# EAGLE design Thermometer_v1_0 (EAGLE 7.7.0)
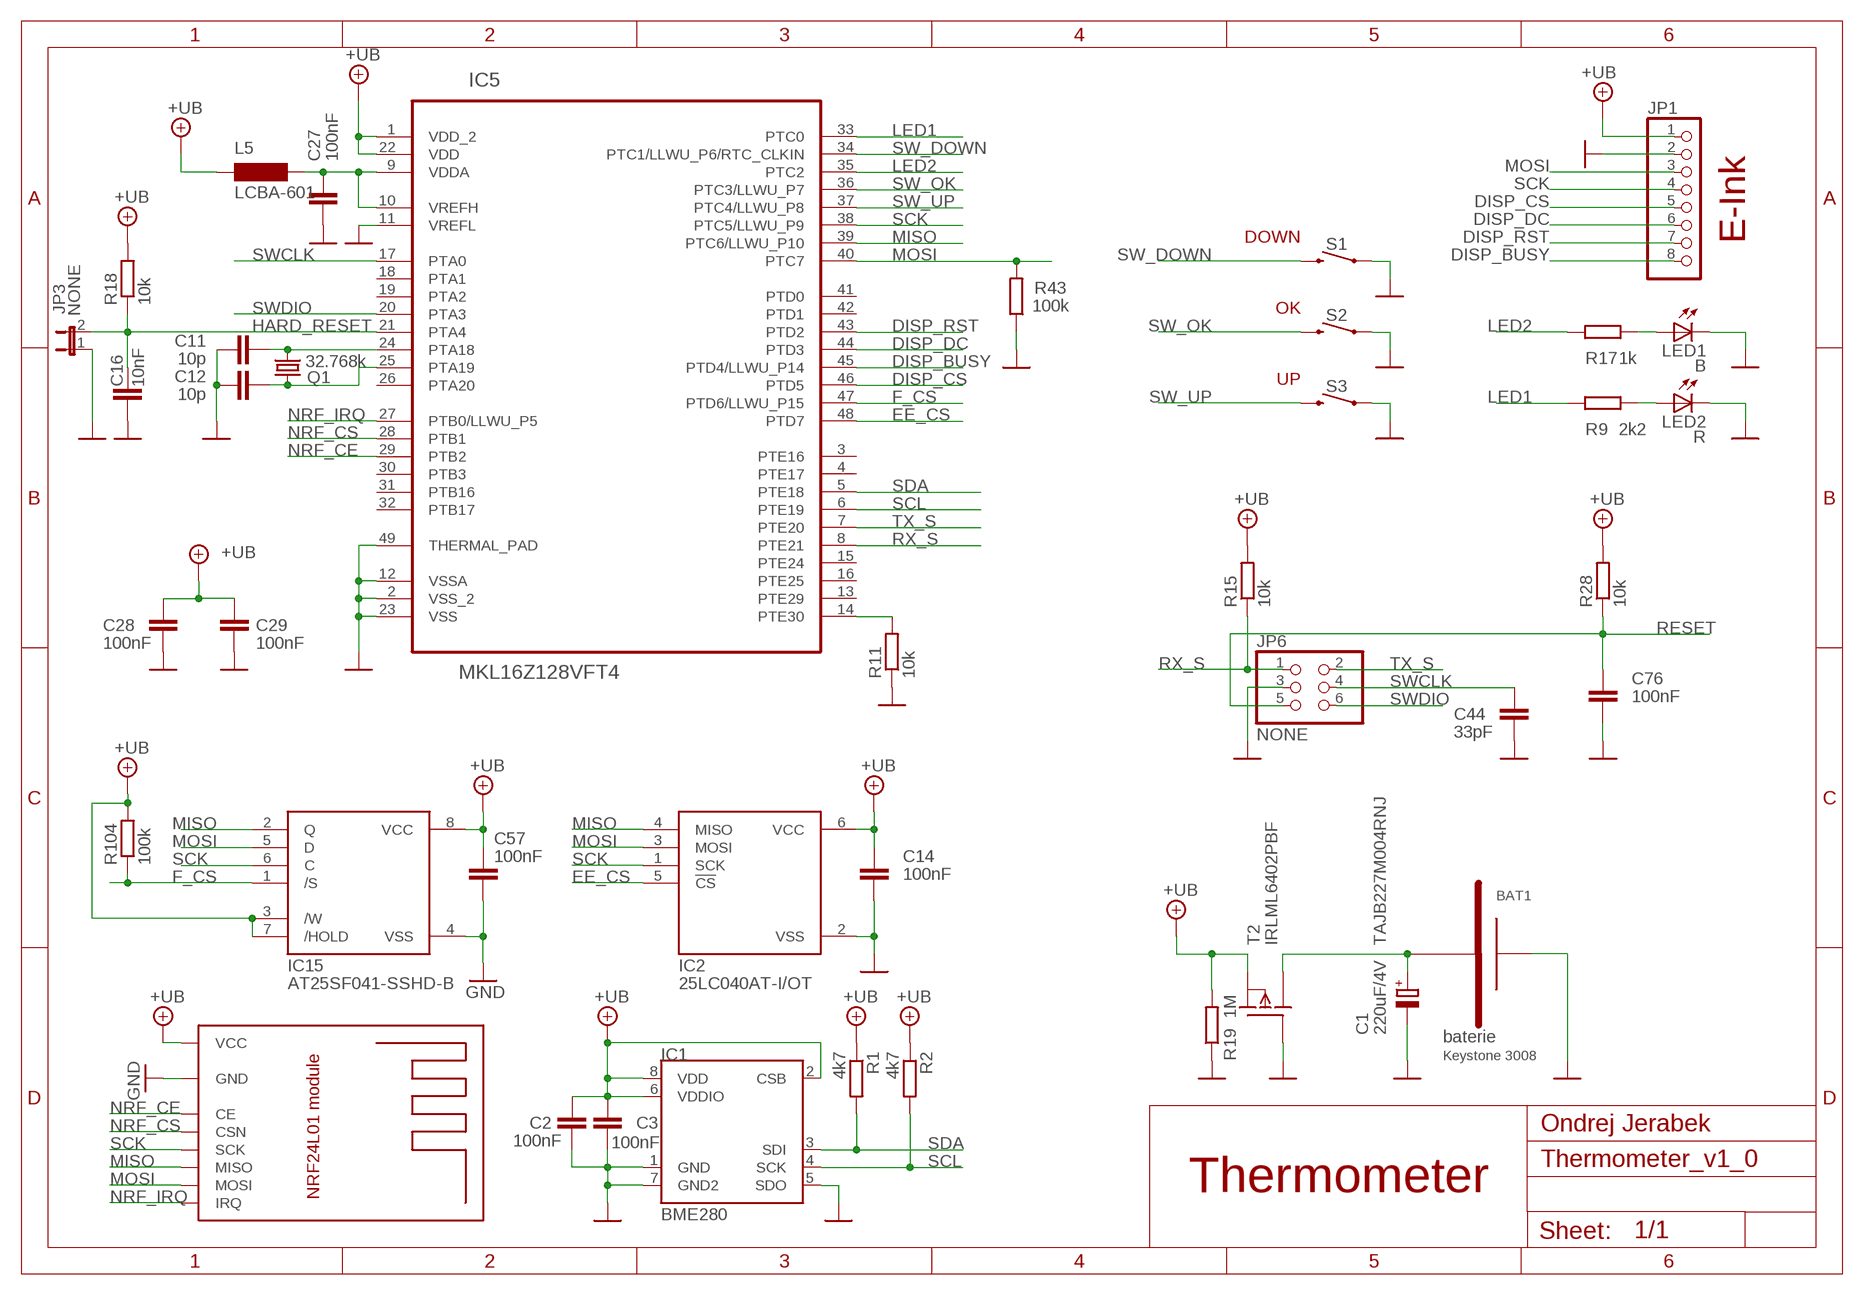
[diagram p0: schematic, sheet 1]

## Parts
BAT1  Keystone 3008  BATT3VSMD  [KEYS3006]
C1  220uF/4V TAJB227M004RNJ  CPOL-EUSMCB  [SMC_B]
C2  100nF  C0603  [C0603]
C3  100nF  C0603  [C0603]
C11  10p  C0603  [C0603]
C12  10p  C0603  [C0603]
C14  100nF  C0603  [C0603]
C16  10nF  C0603  [C0603]
C27  100nF  C0603  [C0603]
C28  100nF  C0603  [C0603]
C29  100nF  C0603  [C0603]
C44  33pF  C0603  [C0603]
C57  100nF  C0603  [C0603]
C76  100nF  C0603  [C0603]
IC1  BME280  BMP280  [BMA150]
IC2  25LC040AT-I/OT  25AA02E48T-I/OT  [EE_SOT23-6]
IC5  MKL16Z128VFT4  [QFN50P700X700X100-49N]
IC15  AT25SF041-SSHD-B  M25P16  [SO-8]
JP1  PINHD-1X8  [1X08]
JP3  NONE  JUMPER2  [M1X2]
JP6  NONE  PINHD-2X3  [2X03]
L5  LCBA-601  [R0603]
LED1  B  LEDCHIPLED_0603  [CHIPLED_0603]
LED2  R  LEDCHIPLED_0603  [CHIPLED_0603]
Q1  32.768k  CRYSTALTC26H  [TC26H]
R1  4k7  R-EU_R0603  [R0603]
R2  4k7  R-EU_R0603  [R0603]
R9  2k2  R0603  [R0603]
R11  10k  R-EU_R0603  [R0603]
R15  10k  R-EU_R0603  [R0603]
R17  1k  R0603  [R0603]
R18  10k  R-EU_R0603  [R0603]
R19  1M  R0603  [R0603]
R28  10k  R-EU_R0603  [R0603]
R43  100k  R0603  [R0603]
R104  100k  R-EU_R0603  [R0603]
S1  B3U-3000PM  MOMENTARY-SWITCH-SPST-SMD-RIGHT-ANGLE  [TACTILE_SWITCH_SMD_RIGHT_ANGLE]
S2  B3U-3000PM  MOMENTARY-SWITCH-SPST-SMD-RIGHT-ANGLE  [TACTILE_SWITCH_SMD_RIGHT_ANGLE]
S3  B3U-3000PM  MOMENTARY-SWITCH-SPST-SMD-RIGHT-ANGLE  [TACTILE_SWITCH_SMD_RIGHT_ANGLE]
T2  IRLML6402PBF  MOSFET-P(SMD)  [SOT23]
U$9  NRF24L01  [NRF24L01MODULE]

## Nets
+UB: C2.1 C3.1 C14.1 C28.1 C29.1 C57.2 IC1.2(CSB) IC1.6(VDDIO) IC1.8(VDD) IC2.6(VCC) IC5.1(VDD_2) IC5.22(VDD) IC15.3(/W) IC15.7(/HOLD) IC15.8(VCC) JP1.1 L5.1 R1.1 R2.1 R15.2 R18.2 R19.2 R28.2 R104.2 T2.2(S) U$9.VCC
DISP_BUSY: IC5.45(PTD4/LLWU_P14) JP1.8
DISP_CS: IC5.46(PTD5) JP1.5
DISP_DC: IC5.44(PTD3) JP1.6
DISP_RST: IC5.43(PTD2) JP1.7
EE_CS: IC2.5(!CS) IC5.48(PTD7)
F_CS: IC5.47(PTD6/LLWU_P15) IC15.1(/S) R104.1
GND: BAT1.N C1.- C2.2 C3.2 C11.1 C12.1 C14.2 C16.2 C27.1 C28.2 C29.2 C44.2 C57.1 C76.2 IC1.1(GND) IC1.5(SDO) IC1.7(GND2) IC2.2(VSS) IC5.2(VSS_2) IC5.11(VREFL) IC5.12(VSSA) IC5.23(VSS) IC5.49(THERMAL_PAD) IC15.4(VSS) JP1.2 JP3.1 JP6.3 LED1.C LED2.C R11.1 R19.1 R43.1 S1.1 S2.1 S3.1 T2.1(G) U$9.GND
HARD_RESET: C16.1 IC5.21(PTA4) JP3.2 R18.1
LED1: IC5.33(PTC0) R9.2
LED2: IC5.35(PTC2) R17.2
MISO: IC2.4(MISO) IC5.39(PTC6/LLWU_P10) IC15.2(Q) U$9.MISO
MOSI: IC2.3(MOSI) IC5.40(PTC7) IC15.5(D) JP1.3 R43.2 U$9.MOSI
N$6: LED2.A R9.1
N$9: C11.2 IC5.24(PTA18) Q1.2
N$10: C12.2 IC5.25(PTA19) Q1.1
N$13: BAT1.POS1(P1) C1.+ T2.3(D)
N$14: LED1.A R17.1
N$18: IC5.14(PTE30) R11.2
N$42: C27.2 IC5.9(VDDA) IC5.10(VREFH) L5.2
NRF_CE: IC5.29(PTB2) U$9.CE
NRF_CS: IC5.28(PTB1) U$9.CSN
NRF_IRQ: IC5.27(PTB0/LLWU_P5) U$9.IRQ
RESET: C76.1 JP6.5 R28.1
RX_S: IC5.8(PTE21) JP6.1 R15.1
SCK: IC2.1(SCK) IC5.38(PTC5/LLWU_P9) IC15.6(C) JP1.4 U$9.SCK
SCL: IC1.4(SCK) IC5.6(PTE19) R2.2
SDA: IC1.3(SDI) IC5.5(PTE18) R1.2
SW_DOWN: IC5.34(PTC1/LLWU_P6/RTC_CLKIN) S1.2
SW_OK: IC5.36(PTC3/LLWU_P7) S2.2
SW_UP: IC5.37(PTC4/LLWU_P8) S3.2
SWCLK: C44.1 IC5.17(PTA0) JP6.4
SWDIO: IC5.20(PTA3) JP6.6
TX_S: IC5.7(PTE20) JP6.2
Unconnected: BAT1.POS2(P2) IC5.3(PTE16) IC5.4(PTE17) IC5.13(PTE29) IC5.15(PTE24) IC5.16(PTE25) IC5.18(PTA1) IC5.19(PTA2) IC5.26(PTA20) IC5.30(PTB3) IC5.31(PTB16) IC5.32(PTB17) IC5.41(PTD0) IC5.42(PTD1)

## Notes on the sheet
- DOWN | E-Ink
- OK
- UP
- baterie
- Ondrej Jerabek
- Thermometer

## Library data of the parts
BAT1 = custom:BATT3V
C1 = rcl:CPOL-EU: POLARIZED CAPACITOR, European symbol
C2 C3 C11 C12 C14 C16 C27-C29 C44 C57 C76 = custom:C
IC1 = #my_lib:BMP280
IC2 = customEE:25AA02E48T-I/OT
IC5 = custom:MKL16Z128VFT4
IC15 = custom:M25P: 64 MBit SPI FLASH
JP1 = pinhead:PINHD-1X8: PIN HEADER
JP3 = q:JUMPER2: JUMPER - 2 Pins
JP6 = pinhead:PINHD-2X3: PIN HEADER
L5 = custom:LCB: LCBA/LCBB/LCBC
LED1 LED2 = led:LED: LED
Q1 = crystal:CRYSTAL: CRYSTAL; OC_FARNELL: unknown; OC_NEWARK: unknown
R1 R2 R11 R15 R18 R28 R104 = rcl:R-EU_: RESISTOR, European symbol
R9 R17 R19 R43 = custom:R
S1-S3 = SparkFun-Switches:MOMENTARY-SWITCH-SPST: Momentary Switch (Pushbutton) - SPST; PROD_ID: COMP-12265
T2 = custom:MOSFET-P
U$9 = #Ondra_lib:NRF24L01

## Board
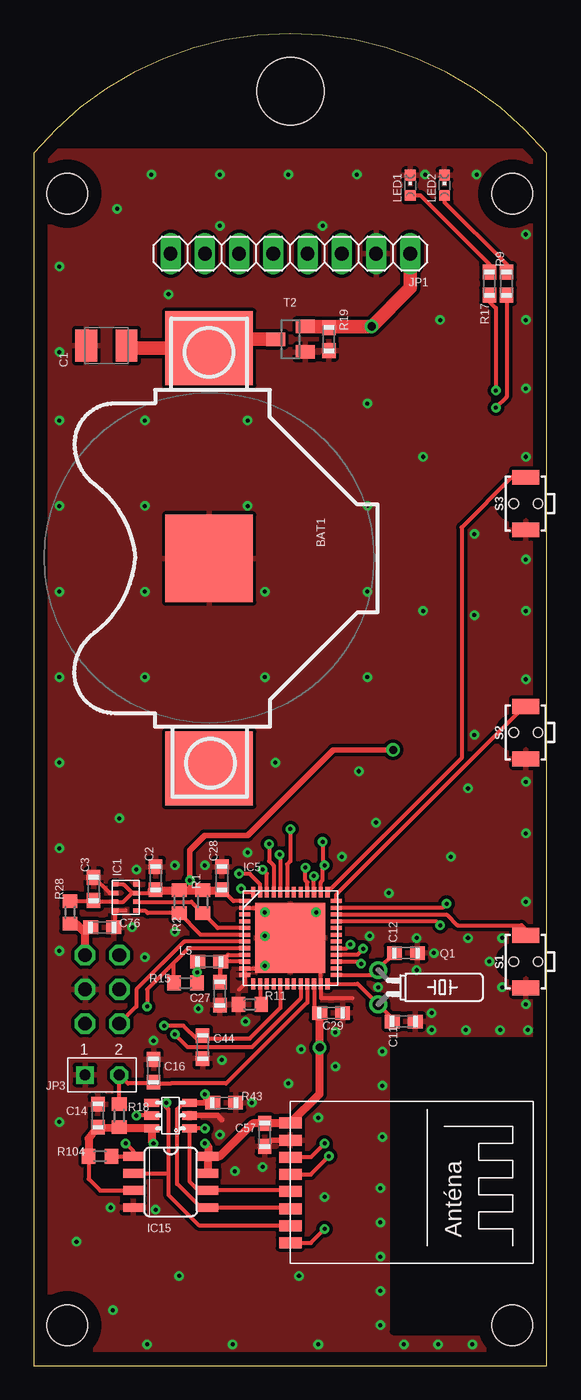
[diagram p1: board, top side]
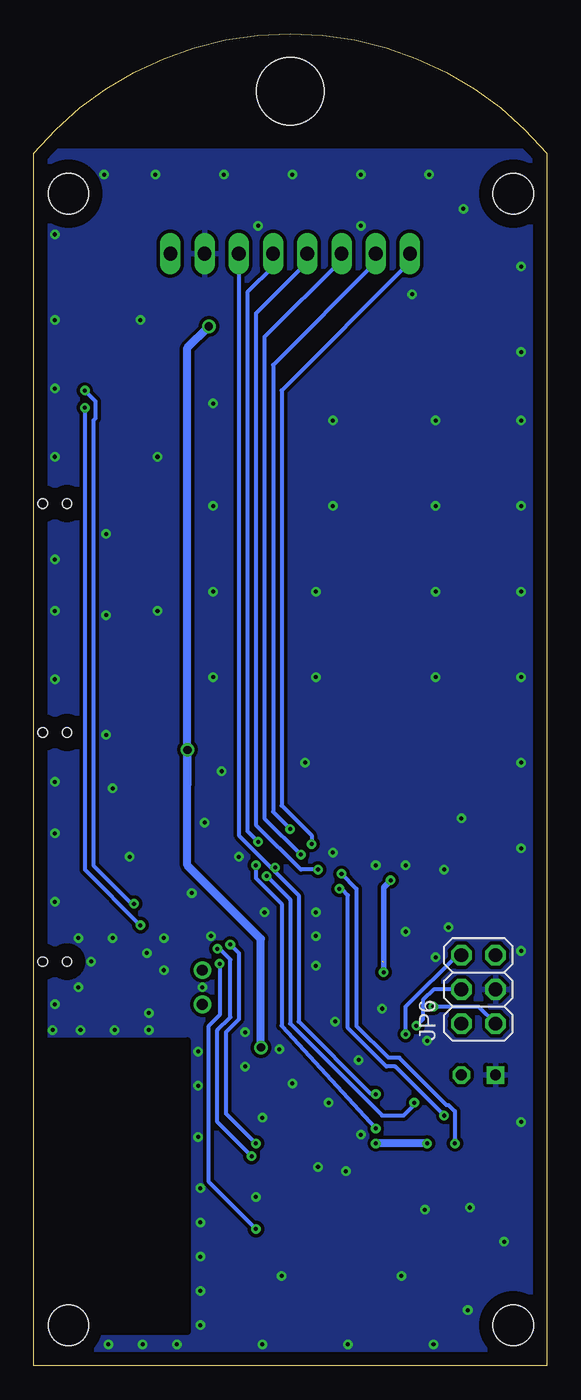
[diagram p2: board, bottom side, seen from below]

Size 38.08 x 98.88 mm. Coordinates in mm from the lower left corner, seen from the top.
Outline: 0,0 38.08,0 38.08,90 arc100 0,90 0,0
Copper layers (1*16): Top 0.035mm / dielectric 1.5mm / Bottom 0.035mm
Design rules "default": minimum track width 10mil, minimum drill 24mil, track to track 8mil, track to pad 8mil, pad to pad 8mil, via to via 8mil, smd to smd 8mil, copper to edge 40mil, drill to drill 8mil, minimum pad ring 10mil, minimum via ring 8mil, stop-mask expansion 4mil, vias tented up to drill 0mil, thermal gap 10mil
Holes 3 mm at 2.5,3 35.5,3 2.5,87 35.5,87
Holes 5 mm at 19.05,94.61
tRestrict: area 26.7,2.5 to 38.1,24.1
bRestrict: area 26.7,2.5 to 38.1,24.1

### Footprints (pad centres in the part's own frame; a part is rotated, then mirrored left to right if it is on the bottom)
KEYS3006 = smd 6.5 x 6.5: N 15,0 | smd 5.5 x 6.5: POS1 -0.6,0; POS2 30.6,0
SMC_B = smd 1.6 x 2.4: + -1.5,0; - 1.5,0
C0603 = smd 1.1 x 1: 1 -0.85,0; 2 0.85,0
BMA150 = smd 0.5 x 0.35: 1 0.8,0.975; 2 0.8,0.325; 3 0.8,-0.325; 4 0.8,-0.975; 5 -0.8,-0.975; 6 -0.8,-0.325; 7 -0.8,0.325; 8 -0.8,0.975
EE_SOT23-6 = smd 0.6 x 1.1: 1 -0.95,-1.4; 2 0,-1.4; 3 0.95,-1.4; 4 0.95,1.4; 5 0,1.4; 6 -0.95,1.4
QFN50P700X700X100-49N = smd 0.8 x 0.3: 1 -3.4,2.75; 2 -3.4,2.25; 3 -3.4,1.75; 4 -3.4,1.25; 5 -3.4,0.75; 6 -3.4,0.25; 7 -3.4,-0.25; 8 -3.4,-0.75; 9 -3.4,-1.25; 10 -3.4,-1.75; 11 -3.4,-2.25; 12 -3.4,-2.75; 25 3.4,-2.75; 26 3.4,-2.25; 27 3.4,-1.75; 28 3.4,-1.25; 29 3.4,-0.75; 30 3.4,-0.25; 31 3.4,0.25; 32 3.4,0.75; 33 3.4,1.25; 34 3.4,1.75; 35 3.4,2.25; 36 3.4,2.75 | smd 0.3 x 0.8: 13 -2.75,-3.4; 14 -2.25,-3.4; 15 -1.75,-3.4; 16 -1.25,-3.4; 17 -0.75,-3.4; 18 -0.25,-3.4; 19 0.25,-3.4; 20 0.75,-3.4; 21 1.25,-3.4; 22 1.75,-3.4; 23 2.25,-3.4; 24 2.75,-3.4; 37 2.75,3.4; 38 2.25,3.4; 39 1.75,3.4; 40 1.25,3.4; 41 0.75,3.4; 42 0.25,3.4; 43 -0.25,3.4; 44 -0.75,3.4; 45 -1.25,3.4; 46 -1.75,3.4; 47 -2.25,3.4; 48 -2.75,3.4 | smd 5.2 x 5.2: 49 0,0
SO-8 = smd 0.66 x 1.5: 1 -1.905,-2.773; 2 -0.635,-2.773; 3 0.635,-2.773; 4 1.905,-2.773; 5 1.905,2.773; 6 0.635,2.773; 7 -0.635,2.773; 8 -1.905,2.773
1X08 = drill 1.016 long: 1 -8.89,0; 2 -6.35,0; 3 -3.81,0; 4 -1.27,0; 5 1.27,0; 6 3.81,0; 7 6.35,0; 8 8.89,0
M1X2 = drill 0.8 pad 1.27 square: 1 1.27,0 | drill 0.8 pad 1.27 octagon: 2 -1.27,0
2X03 = drill 1.016 octagon: 1 -2.54,-1.27; 2 -2.54,1.27; 3 0,-1.27; 4 0,1.27; 5 2.54,-1.27; 6 2.54,1.27
R0603 = smd 1.1 x 1: 1 -0.85,0; 2 0.85,0
CHIPLED_0603 = smd 0.8 x 0.8: A 0,-0.75; C 0,0.75
TC26H = drill 0.813: 1 -1.27,0; 2 1.27,0
R0603' = smd 1 x 1.1: 1 -0.85,0; 2 0.85,0
TACTILE_SWITCH_SMD_RIGHT_ANGLE = smd 1.1 x 2: 1 -1.95,0; 2 1.95,0 | hole 0.7: 0,0.9; 0,-0.9
SOT23 = smd 1 x 1.4: 1 -0.95,-1.1; 2 0.95,-1.1; 3 0,1.1
NRF24L01MODULE = smd 1.676 x 0.813: CE 0,7.86; CSN 0,6.59; GND 0,9.13; IRQ 0,1.51; MISO 0,2.78; MOSI 0,4.05; SCK 0,5.32; VCC 0,10.4

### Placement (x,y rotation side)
BAT1  13.02,74.93 270 top
C1  5.4,75.72 180 top
C2  9.05,36.2 90 top
C3  4.45,35.4 90 top
C11  27.46,25.56 180 top
C12  27.62,30.64 180 top
C14  4.76,18.57 90 top
C16  8.89,21.91 90 top
C27  13.81,27.62 90 top
C28  13.97,36.2 90 top
C29  22.07,26.19 0 top
C44  12.54,23.65 270 top
C57  17.14,17.14 90 top
C76  5.08,32.54 0 top
IC1  6.83,34.77 0 top
IC2  10.16,18.57 90 top
IC5  19.05,31.75 0 top
IC15  10.16,13.65 270 top
JP1  19.05,82.55 180 top
JP3  5.08,21.59 180 top
JP6  5.08,27.94 90 bottom
L5  13.02,30 0 top
LED1  27.94,87.63 0 top
LED2  30.48,87.63 0 top
Q1  25.56,28.1 270 top
R1  4k7  [R0603']  12.54,34.45 270 top
R2  4k7  [R0603']  10.79,34.45 270 top
R9  35.08,80.33 270 top
R11  10k  [R0603']  16.03,26.83 0 top
R15  10k  [R0603']  11.27,28.42 0 top
R17  33.81,80.33 270 top
R18  10k  [R0603']  6.35,18.57 270 top
R19  21.91,76.2 90 top
R28  10k  [R0603']  2.7,33.66 90 top
R43  14.13,19.53 180 top
R104  100k  [R0603']  4.92,15.56 180 top
S1  36.51,30 90 top
S2  36.51,47 90 top
S3  36.51,64 90 top
T2  19.05,76.2 90 top
U$9  19.05,7.62 0 top

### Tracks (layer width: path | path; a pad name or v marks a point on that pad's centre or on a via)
+UB  (via drill 0.3, 0.6)  (1 unrouted)
  Top 0.305: IC5.22 20.8,26.61 C29.1 | IC5.1 14.81,34.5 C28.1 | 8.75,35.3 C2.1 8.5,35.09 IC1.2 | IC1.2 7.29,35.09 6.67,35.72 6.05,35.72 IC1.8 | IC1.2 7.31,35.09 6.66,34.44 IC1.6 4.53,34.44 C3.1 4.42,34.51 R28.2 | R104.2 4.07,13.87 4.92,13.02 IC15.3 | 8.76,16.64 v8.89,16.51 | v11.59,36.04 11.59,35.46 11.43,35.3
  Top 0.406: 6.45,17.62 R18.2 6.25,17.62 | U$9.VCC 19.05,18 | 12.12,29.96 v12.12,29.21 | v12.12,29.21 R15.2 | R2.1 10.9,35.4 | v12.12,29.21 12.17,29.26 | v11.59,36.04 11.59,38.26 12.7,39.37 15.88,39.37 22.23,45.72 v26.67,45.72
  Top 0.61: 6.45,17.62 IC2.6 8.76,16.64 | IC15.7 IC15.8 | 8.75,35.3 R2.1 11.43,35.3 R1.1 13.92,35.3 C28.1 | 6.25,17.62 C14.1 4.07,16.85 R104.2 | 19.05,18 C57.2 16.25,18 13.81,15.56 IC15.8 | v12.7,16.51 12.93,16.28 IC15.8 | U$9.VCC 21.22,20.19 v21.22,23.62 C29.1
  Top 1.016: T2.2 21.81,77.15 | 21.81,77.15 R19.2 | JP1.1 27.94,80.01 v25.08,77.15 21.81,77.15
  Bottom 0.406: v11.59,36.04 12.12,35.5 v12.12,29.21
  Bottom 0.61: v8.89,16.51 v12.7,16.51 | v21.22,23.62 21.22,31.69 26.67,37.15 v26.67,45.72 | v26.67,45.72 26.67,43.18 | v26.67,45.72 26.67,75.56 v25.08,77.15
DISP_BUSY  (via drill 0.3)
  Top 0.305: v17.46,38.73 17.46,37.47 17.8,37.13 IC5.45
  Bottom 0.305: JP1.8 10.16,81.92 19.68,72.39 19.68,41.59 17.46,39.37 v17.46,38.73
DISP_CS  (via drill 0.3)
  Top 0.305: IC5.46 17.3,36.52 v16.99,36.83
  Bottom 0.305: JP1.5 17.78,81.92 21.59,78.11 21.59,40.16 18.26,36.83 v16.99,36.83
DISP_DC  (via drill 0.3)
  Top 0.305: v18.26,37.94 18.3,37.9 IC5.44
  Bottom 0.305: JP1.6 15.24,82.07 20.95,76.36 20.95,40.64 v18.26,37.94
DISP_RST  (via drill 0.3)
  Top 0.305: IC5.43 18.8,37.22 19.05,37.47 v19.05,39.85
  Bottom 0.305: JP1.7 12.7,81.92 20.32,74.3 20.32,41.12 v19.05,39.85
EE_CS  (via drill 0.3)
  Top 0.305: IC5.48 15.65,35.15 v15.4,35.4 | IC2.5 v7.62,18.57
  Bottom 0.305: v15.4,35.4 15.24,35.4 14.76,34.92 14.76,25.08 11.91,22.23 11.27,22.23 v7.62,18.57
F_CS  (via drill 0.3)
  Top 0.305: v6.83,16.51 7.39,15.95 IC15.1 R104.1 | IC5.47 16.8,35.75 16.03,36.51 v15.24,36.51
  Bottom 0.305: v6.83,16.51 6.83,18.89 7.3,19.37 7.46,19.37 10.95,22.86 11.75,22.86 14.13,25.24 14.13,35.4 v15.24,36.51
GND  (via drill 0.3)
  Top 0.305: IC5.2 16.8,34 v17.14,33.66 | 17.94,30.32 17.12,29.5 IC5.11 IC5.12 15.65,28.35 15.24,27.94 | 20.32,30.64 21.3,29.66 IC5.23 21.3,27.3 23.65,27.3 | IC1.7 5.63,35.09 C3.2 | C76.2 6.03,32.62 IC1.5 6.8,33.79 6.83,33.81
  Top 0.406: U$9.GND 17.6,16.75 C57.1 | IC2.2 13.65,18.57 13.97,18.26
  other vias: 6.35,40.64 17.14,29.69 17.14,31.91 32.54,1.59 30,1.59 27.46,1.59 25.72,3.02 25.72,5.56 25.72,8.1 25.72,10.64 25.72,13.18 25.88,16.99 25.88,20.8 25.88,23.34 29.53,24.92 29.53,26.19 32.07,24.92 34.61,24.92 36.67,24.92 36.51,26.83 34.77,28.1 34.77,31.75 33.81,30 32.23,31.75 28.42,31.75 29.69,30.64 28.42,29.37 24.92,31.91 22.38,24.77 22.38,22.23 21.11,18.41 19.84,23.5 16.19,19.53 13.81,17.14 18.89,20.95 13.97,22.7 15.72,25.56 12.22,26.51 8.89,24.13 21.59,12.54 16.99,14.76 14.92,14.45 9.05,11.59 5.71,11.75 19.68,6.67 10.79,6.67 3.17,9.21 1.91,18.1 10.48,32.23 8.26,30.32 7.3,32.54 10.48,37.15 12.7,37.15 15.88,38.1 22.86,37.78 25.4,40.32 24.13,44.13 36.51,34.45 36.51,39.53 36.51,43.34 36.51,50.96 36.51,56.04 36.51,59.85 36.51,67.47 36.51,72.55 36.51,77.63 36.51,83.98 32.86,88.42 29.05,88.42 23.97,88.42 18.89,88.42 13.81,88.42 8.73,88.42 6.19,85.88 1.91,30.8 1.91,38.42 1.91,44.77 1.91,51.12 1.91,57.47 1.91,63.82 1.91,70.17 1.91,75.25 1.91,81.6 8.26,70.17 15.88,70.17 8.26,63.82 15.88,63.82 8.26,57.47 17.14,57.47 8.26,51.12 17.14,51.12 24.77,51.12 24.77,57.47 24.77,63.82 24.77,71.44 17.94,44.77 20.95,33.66 30.96,37.78 32.23,42.86 32.7,46.83 32.7,55.72 32.7,61.75 28.89,67.47 30.16,77.63 10,79.53 21.43,84.61 13.81,84.61 28.89,56.04 26.35,35.08 7.62,36.83 21.11,1.59 14.76,1.59 8.41,1.59 5.87,4.13 25.56,28.1
  pour Top (isolate 0.254): 0,90.17 38.1,90.17 38.1,0 0,0
  pour Bottom (isolate 0.254): 0,90.17 38.1,90.17 38.1,0 0,0
HARD_RESET
  Top 0.305: IC5.21 20.3,26.97 14.29,20.95 10.16,20.95 8.89,20.95 | R18.1 JP3.2 6.99,20.95 8.89,20.95 | C16.1 8.89,20.95
LED1  (via drill 0.3)
  Top 0.305: R9.2 35.08,71.91 v34.29,71.12 | v30.16,32.7 29.86,33 IC5.33
  Bottom 0.305: v34.29,71.12 34.29,36.83 v30.16,32.7
LED2  (via drill 0.3)
  Top 0.305: v34.29,72.39 34.29,78.53 33.81,79 R17.2 | v30.64,34.29 30.35,34 IC5.35
  Bottom 0.305: v34.29,72.39 33.5,71.6 33.5,70.33 33.66,70.17 33.66,37.15 30.96,34.45 v30.64,34.29
MISO  (via drill 0.3)
  Top 0.305: IC5.39 v20.8,36.35 | IC2.4 9.53,19.52 | 9.53,19.52 10,19.05 10,14.29 | 10,14.29 10,12.7 12.3,10.4 U$9.MISO | IC15.2 10,14.29 | 9.53,19.52 9.53,19.53 v9.84,19.53
  Bottom 0.305: v20.8,36.35 19.05,34.61 19.05,25.4 12.22,18.57 10.64,18.57 9.84,19.37 v9.84,19.53
MOSI  (via drill 0.3)
  Top 0.305: IC5.40 20.3,35.9 20.16,36.04 v20.16,36.99 | IC2.3 11.11,19.52 10.64,19.05 10.64,13.49 12.38,11.75 IC15.5 18.97,11.75 | v12.7,20.16 12.7,19.53
  Top 0.406: R43.2 12.7,19.53 IC2.3
  Top 0.61: U$9.MOSI 18.97,11.75
  Bottom 0.305: JP1.3 22.86,39.37 20.48,36.99 | 20.32,36.99 v20.16,36.99 20.48,36.99 | 20.48,36.99 18.41,34.92 18.41,25.56 13.02,20.16 v12.7,20.16
N$6
  Top 0.305: LED2.A 30.48,86.36 35.08,81.76 R9.1
N$9
  Top 0.305: IC5.24 24.04,28.35 Q1.2 26.59,25.8 C11.2
N$10
  Top 0.305: 25.35,29.16 Q1.1 | Q1.1 25.56,29.45 C12.2 | IC5.25 25.19,29 Q1.1
N$13
  Top 1.016: C1.+ 7.09,75.53 BAT1.POS1 12.7,74.93 13.97,76.2 T2.3
N$14
  Top 0.305: LED1.A 28.69,86.88 33.81,81.76 R17.1
N$18
  Top 0.305: IC5.14 16.8,26.91 R11.2
N$42
  Top 0.305: IC5.9 14.41,30.5 13.91,30 | L5.2 C27.2 13.81,29.9 13.91,30 | IC5.10 13.91,30
NRF_CE  (via drill 0.3)
  Top 0.305: IC5.29 23.22,31 v23.5,31.27 | v21.59,16.51 20.56,15.48 U$9.CE
  Bottom 0.305: v23.5,31.27 22.86,30.64 22.86,25.72 23.81,24.77 23.81,18.73 v21.59,16.51
NRF_CS  (via drill 0.3)
  Top 0.305: U$9.CSN 20.56,14.21 v21.91,15.56 | IC5.28 23.99,30.5 v24.45,30.96
  Bottom 0.305: v21.91,15.56 24.45,18.1 24.45,24.92 23.5,25.88 23.5,30.16 24.29,30.96 v24.45,30.96
NRF_IRQ  (via drill 0.3)
  Top 0.305: U$9.IRQ 20.56,9.13 v21.59,10.16 | IC5.27 24.13,30 v24.29,29.84
  Bottom 0.305: v21.59,10.16 25.08,13.65 25.08,25.24 24.29,26.04 v24.29,29.84
RESET
  Top 0.61: JP6.5 3.81,32.15 | 3.81,32.15 C76.1 | R28.1 3.15,32.8 3.81,32.15
RX_S  (via drill 0.3)
  Top 0.305: IC5.8 11.47,31 10.4,29.92 | 10.4,29.92 8.41,27.94 v8.41,26.67 | R15.1 10.4,28.44 10.4,29.92
  Bottom 0.305: v8.41,26.67 5.08,26.67 JP6.1
SCK  (via drill 0.3)
  Top 0.305: v21.43,38.89 21.43,36.99 | IC5.38 21.3,35.91 21.43,36.04 21.43,36.99 | 18.97,13.02 IC15.6 12.22,13.02 11.59,13.65 11.59,17.59 IC2.1 12.07,17.62 v12.7,17.62 | 21.43,36.99 v21.59,37.15
  Top 0.61: U$9.SCK 18.97,13.02
  Bottom 0.305: JP1.4 20.32,81.6 22.23,79.69 22.23,39.69 v21.43,38.89 | v21.59,37.15 21.59,36.2 19.68,34.29 19.68,25.24 v12.7,17.62
SCL
  Top 0.305: IC5.6 12.39,32 R2.2 8.45,33.6 8.26,33.79 IC1.4
SDA
  Top 0.305: IC5.5 13.64,32.5 R1.2 11.7,34.44 IC1.3
SW_DOWN
  Top 0.305: IC5.34 30.64,33.5 31.43,32.7 36.2,32.7 36.51,32.38 S1.2
SW_OK
  Top 0.305: IC5.36 22.45,34.99 36.41,48.95 S2.2
SW_UP
  Top 0.305: S3.2 35.47,65.95 31.75,62.23 31.75,45.1 IC5.37
SWCLK  (via drill 0.3)
  Top 0.305: IC5.17 18.3,26.55 16.03,24.29 13.97,24.29 12.76,24.29 | v9.68,25.24 11.11,25.24 12.06,24.29 12.76,24.29 | C44.1 12.76,24.29
  Bottom 0.305: JP6.4 8.41,27.94 9.21,27.15 9.21,25.72 v9.68,25.24
SWDIO  (via drill 0.3)
  Top 0.305: IC5.20 19.8,27.26 16.19,23.65 11.43,23.65 v10.48,24.61
  Bottom 0.305: JP6.6 6.67,30.48 10.48,26.67 v10.48,24.61
TX_S
  Top 0.305: IC5.7 11.18,31.5 7.62,27.94 7.62,26.67 JP6.2

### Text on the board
bStop: e-Paper Smart Thermometer v1.0 / Ondrej Jerabek 2018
